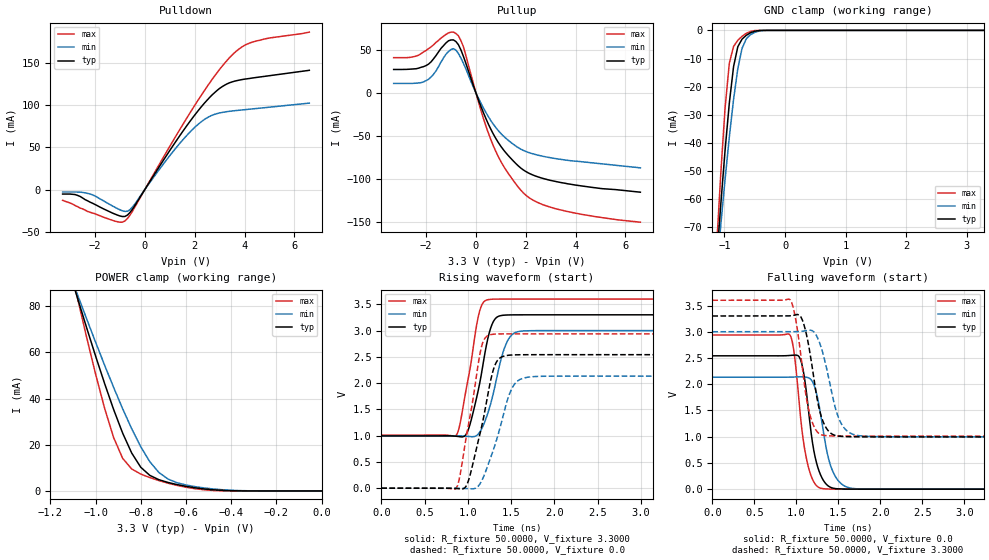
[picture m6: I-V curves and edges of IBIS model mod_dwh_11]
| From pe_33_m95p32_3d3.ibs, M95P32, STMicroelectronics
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|   Model mod_dwh_11
[Model]   mod_dwh_11
Model_type I/O
Polarity   Non-Inverting
Vinl   =   1.000V
Vinh   =   2.300V
Vmeas  =   1.650V
Cref   =   30pF
C_comp   1.607pF   1.535pF   1.683pF
[Model Spec]
Vinl   1.000V  0.900V  1.080V  | <- for Vcc = 3.3V, 3.0V, 3.6V
Vinh   2.300V  2.100V  2.520V  | <- for Vcc = 3.3V, 3.0V, 3.6V
Vmeas  1.650V  1.500V  1.800V  | <- for Vcc = 3.3V, 3.0V, 3.6V
[Temperature Range]   25.0000   0.1050k   -40.0000
[Voltage Range]   3.3000V   3.0000V   3.6000V
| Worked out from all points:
|   slope of the pulldown table from 0 to 0.495 V, typ, clamps not added: 21.3 ohm
|   slope of the pullup table from 0 to 0.495 V, typ, clamps not added: 13.8 ohm
|   GND clamp passes 1 mA (typ) near -0.58 V on its own axis
|   POWER clamp passes 1 mA (typ) near -0.53 V on its own axis
|   rising waveform, R_fixture 50.0000, V_fixture 3.3000: 20-80 % time 167ps typ, 185ps min, 156ps max; typ from 0.995 V to 3.3 V
|   rising waveform, R_fixture 50.0000, V_fixture 0.0: 20-80 % time 197ps typ, 233ps min, 174ps max; typ from 0 V to 2.54 V
|   falling waveform, R_fixture 50.0000, V_fixture 0.0: 20-80 % time 135ps typ, 155ps min, 128ps max; typ from 2.54 V to 0 V
|   falling waveform, R_fixture 50.0000, V_fixture 3.3000: 20-80 % time 149ps typ, 180ps min, 137ps max; typ from 3.3 V to 0.995 V
[Pulldown]
|Voltage   I(typ)   I(min)   I(max)
-3.3V     -5.4mA     -3mA       -12.82mA
-2.8V     -6mA       -3mA       -19mA
-2.2V     -15mA      -5.3mA     -27mA
-1.2V     -29.2mA    -21.1mA    -37.6mA
-800mV    -32.02mA   -26.05mA   -37.38mA
-500mV    -23.51mA   -20.95mA   -25.93mA
1V        46.29mA    40.16mA    51.22mA
2V        88.39mA    73.76mA    99.86mA
2.6V      109.4mA    86.84mA    126.6mA
3.4V      126.8mA    92.92mA    156.7mA
4.3V      132.4mA    95.71mA    175mA
6.6V      141.6mA    102.6mA    187mA
[Pullup]
|Voltage   I(typ)   I(min)   I(max)
-3.3V     26.92mA    10.78mA    40.59mA
-2.5V     27.54mA    10.88mA    41.66mA
-2V       31.42mA    14.02mA    48.88mA
-1.1V     60.1mA     47.6mA     69.21mA
-800mV    59.17mA    49.22mA    68.51mA
-500mV    42.04mA    34.06mA    53.16mA
200mV     -15.63mA   -11.97mA   -20.15mA
700mV     -47.77mA   -36.41mA   -61.37mA
1.2V      -69.34mA   -52.57mA   -89.03mA
1.9V      -89.18mA   -66.58mA   -115.7mA
3.2V      -102.6mA   -76.15mA   -134.1mA
6.6V      -115mA     -86.85mA   -149.7mA
[GND_clamp]
|Voltage   I(typ)   I(min)   I(max)
-3.3V     -807.6mA   -672mA     -1.053A
-1.13V    -81.94mA   -85.75mA   -76.94mA
-1.06V    -61.58mA   -68.96mA   -50.51mA
-990mV    -42.58mA   -52.9mA    -27.53mA
-920mV    -25.81mA   -37.91mA   -11.64mA
-850mV    -12.88mA   -24.52mA   -5.709mA
-780mV    -5.82mA    -13.61mA   -3.523mA
-710mV    -3.106mA   -6.377mA   -2.091mA
-640mV    -1.742mA   -2.986mA   -1.046mA
-500mV    -309.6uA   -721.8uA   -69.16uA
-290mV    -791nA     -10.61uA   -17.06nA
3.28V     561.4pA    18.21uA    173.1pA
[POWER_clamp]
|Voltage   I(typ)   I(min)   I(max)
-3.28V    853.2mA    705.5mA    1.123A
-1.08V    83.64mA    85.1mA     83.66mA
-1V       58.53mA    64.51mA    50.75mA
-960mV    46.59mA    54.53mA    35.87mA
-920mV    35.3mA     44.85mA    23.13mA
-880mV    25.04mA    35.59mA    14.12mA
-840mV    16.42mA    26.93mA    9.512mA
-800mV    10.26mA    19.14mA    7.302mA
-720mV    4.876mA    8.001mA    4.493mA
-640mV    2.758mA    3.578mA    2.397mA
-400mV    94.29uA    284.7uA    12.64uA
0V        840.7pA    17.31nA    345.8pA
[Ramp]
| variable   typ   min   max
dV/dt_r   1.5248/0.2164n   1.2991/0.2403n   1.7626/0.1812n
dV/dt_f   1.3827/0.1694n   1.2128/0.2091n   1.5533/0.1622n
R_load = 50.0000
[Rising Waveform]
R_fixture= 50.0000
V_fixture= 3.3000
V_fixture_min= 3.0000
V_fixture_max= 3.6000
|time   V(typ)   V(min)   V(max)
0s        995.5mV    997.2mV    1.011V
864ps     988.9mV    997.8mV    1.002V
912ps     979.5mV    995.5mV    1.245V
1.008ns   1.127V     985mV      2.12V
1.136ns   1.991V     1.063V     3.371V
1.232ns   2.858V     1.436V     3.588V
1.312ns   3.217V     1.934V     3.599V
1.424ns   3.294V     2.672V     3.6V
1.584ns   3.3V       2.981V     3.6V
6ns       3.3V       3V         3.6V
[Rising Waveform]
R_fixture= 50.0000
V_fixture= 0.0
V_fixture_min= 0.0
V_fixture_max= 0.0
|time   V(typ)   V(min)   V(max)
0s        4.444nV    483.6nV    774.5pV
864ps     -5.061mV   869.7uV    -1.841mV
912ps     -12.78mV   -492.7uV   264mV
1.008ns   149.2mV    -8.221mV   1.222V
1.152ns   1.117V     115.5mV    2.655V
1.248ns   1.93V      511.3mV    2.916V
1.344ns   2.436V     985mV      2.936V
1.488ns   2.534V     1.823V     2.938V
1.664ns   2.541V     2.104V     2.938V
6ns       2.541V     2.133V     2.938V
[Falling Waveform]
R_fixture= 50.0000
V_fixture= 0.0
V_fixture_min= 0.0
V_fixture_max= 0.0
|time   V(typ)   V(min)   V(max)
0s        2.541V     2.133V     2.938V
920ps     2.548V     2.135V     2.949V
968ps     2.553V     2.137V     2.663V
1.048ns   2.478V     2.141V     1.408V
1.112ns   1.95V      2.135V     649.3mV
1.208ns   737.4mV    1.996V     137.7mV
1.288ns   274mV      1.44V      18.64mV
1.432ns   21.11mV    346.3mV    1.627mV
1.656ns   1.059mV    17.74mV    69.28uV
6ns       1.679uV    2.784uV    1.697uV
[Falling Waveform]
R_fixture= 50.0000
V_fixture= 3.3000
V_fixture_min= 3.0000
V_fixture_max= 3.6000
|time   V(typ)   V(min)   V(max)
0s        3.3V       3V         3.6V
928ps     3.304V     2.999V     3.607V
1.008ns   3.328V     3.002V     3.09V
1.088ns   3.148V     3.013V     2.089V
1.184ns   2.38V      3.024V     1.299V
1.248ns   1.72V      2.901V     1.095V
1.312ns   1.314V     2.615V     1.03V
1.504ns   1.011V     1.355V     1.012V
1.712ns   997.1mV    1.029V     1.011V
6ns       995.5mV    997.2mV    1.011V
